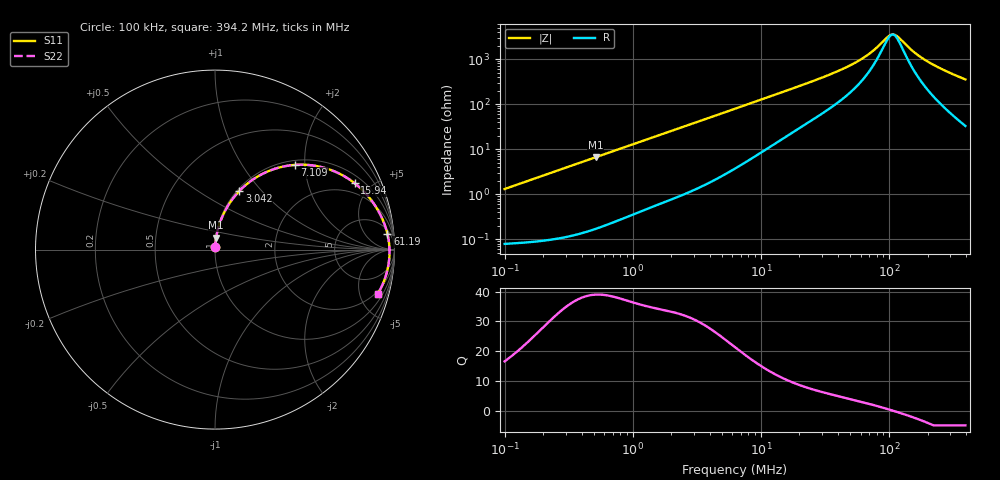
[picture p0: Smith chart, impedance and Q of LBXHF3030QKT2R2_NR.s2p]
! LBXHF3030QKT2R2_NR  S-PARAMETER MODEL  ( General Type )
! Model Generated by TAIYO YUDEN Corporation (http://www.ty-top.com)
! Version 1.0
! TAIYO YUDEN Control No. 210113NI43SB-FBB
! Copyright(c) 2021 TAIYO YUDEN CO.,LTD. All Rights Reserved.
! Product Description (link to TY-COMPAS)
! https://ds.yuden.co.jp/TYCOMPAS/or/detail?pn=LBXHF3030QKT2R2MNR&u=M
! Products Name : Inductors
! Characteristics :
!  Inductance : 2.2 uH , SRF(min) : 60 MHz , DC Resistance(max) : 0.072 Ohm
!  Rated Current : Saturation :1500 mA , Temp Rise : 1400 mA
!  Case Size : 3.0 x 3.0 / 0.118 x 0.118 [mm/inch] , Thickness : 1.5 / 0.059 [mm/inch]
!  (Conditions: Temperature = 25 degC , DC Bias Current/Voltage = 0A / 0V)
! External Node Assignments :
!  1  o---GGG---o  2
! GND o---------o GND
! Frequency Range : 0.1MHz  -  394.189695MHz  [ 402 STEP ]
# MHz S RI R 50
! Freq[MHz].  S11 Real  S11 Imag  S21 Real  S21 Imag  S12 Real  S12 Imag  S22 Real  S22 Imag
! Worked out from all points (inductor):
!   401 points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, 100 kHz to 394.2 MHz, reference 50 ohm
!   read as one part in series: L = 2.07 uH near 104.2 kHz
!   highest Q = 39 at 513 kHz (marker M1), where L = 2.05 uH
!   self-resonance near 106.5 MHz
!   S11 on the Smith chart (normalised r, x): 100 kHz: 1.00, +0.03; 3.042 MHz: 1.03, +0.77; 7.109 MHz: 1.09, +1.78; 15.94 MHz: 1.39, +3.99; 61.19 MHz: 8, +19; 394.2 MHz: 1.65, -7.03
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0.1  0.000956 0.013  0.999 -0.013  0.999 -0.013  0.000956 0.013
0.400203  0.00401 0.0514  0.996 -0.0514  0.996 -0.0514  0.00401 0.0514
0.513041  0.00603 0.0656  0.994 -0.0656  0.994 -0.0656  0.00603 0.0656
0.935062  0.0173 0.1173  0.9827 -0.1173  0.9827 -0.1173  0.0173 0.1173
1.601627  0.045 0.1932  0.955 -0.1932  0.955 -0.1932  0.045 0.1932
3.042485  0.1363 0.3271  0.8637 -0.3271  0.8637 -0.3271  0.1363 0.3271
4.325595  0.2368 0.4067  0.7632 -0.4067  0.7632 -0.4067  0.2368 0.4067
6.278453  0.3886 0.4645  0.6114 -0.4645  0.6114 -0.4645  0.3886 0.4645
7.108668  0.4463 0.4721  0.5537 -0.4721  0.5537 -0.4721  0.4463 0.4721
10.10661  0.6096 0.4554  0.3904 -0.4554  0.3904 -0.4554  0.6096 0.4554
15.93564  0.7789 0.3692  0.2211 -0.3692  0.2211 -0.3692  0.7789 0.3692
25.12657  0.881 0.2614  0.119 -0.2614  0.119 -0.2614  0.881 0.2614
42.15653  0.9399 0.1531  0.0601 -0.1531  0.0601 -0.1531  0.9399 0.1531
61.18875  0.9608 0.0873  0.0392 -0.0873  0.0392 -0.0873  0.9608 0.0873
75.26  0.9674 0.0539  0.0326 -0.0539  0.0326 -0.0539  0.9674 0.0539
100.5574  0.972 0.00887  0.028 -0.00887  0.028 -0.00887  0.972 0.00887
106.9995  0.9724 -0.000688  0.0276 0.000688  0.0276 0.000688  0.9724 -0.000688
113.8543  0.9725 -0.0103  0.0275 0.0103  0.0275 0.0103  0.9725 -0.0103
158.5542  0.9694 -0.0631  0.0306 0.0631  0.0306 0.0631  0.9694 -0.0631
211.8495  0.9605 -0.1141  0.0395 0.1141  0.0395 0.1141  0.9605 -0.1141
288.979  0.9412 -0.1766  0.0588 0.1766  0.0588 0.1766  0.9412 -0.1766
394.1897  0.9061 -0.2489  0.0939 0.2489  0.0939 0.2489  0.9061 -0.2489
